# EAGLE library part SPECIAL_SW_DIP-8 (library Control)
DIP SWITCH
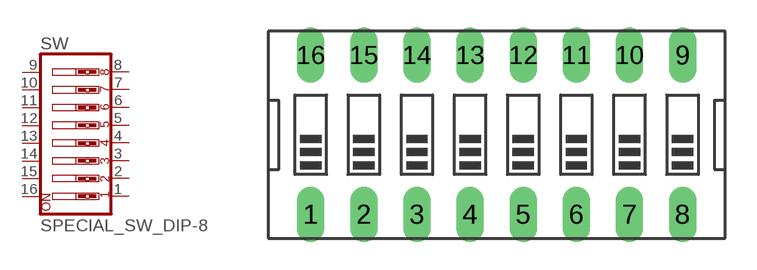
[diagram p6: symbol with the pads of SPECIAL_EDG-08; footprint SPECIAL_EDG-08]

Designator prefix SW

## SPECIAL_SW_DIP-8  [SPECIAL_EDG-08]
1  1  pas
2  2  pas
3  3  pas
4  4  pas
5  5  pas
6  6  pas
7  7  pas
8  8  pas
9  9  pas
10  10  pas
11  11  pas
12  12  pas
13  13  pas
14  14  pas
15  15  pas
16  16  pas

## Footprint SPECIAL_EDG-08 (pad centres in mm)
DIP SWITCH
drill 0.813 long: 1 -8.89,-3.81; 2 -6.35,-3.81; 3 -3.81,-3.81; 4 -1.27,-3.81; 5 1.27,-3.81; 6 3.81,-3.81; 7 6.35,-3.81; 8 8.89,-3.81; 9 8.89,3.81; 10 6.35,3.81; 11 3.81,3.81; 12 1.27,3.81; 13 -1.27,3.81; 14 -3.81,3.81; 15 -6.35,3.81; 16 -8.89,3.81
